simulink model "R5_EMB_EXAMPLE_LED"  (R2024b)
settings: Solver=FixedStepDiscrete  StartTime=0.0  StopTime=S  FixedStep=T  RelTol=1e-3  EnableMultiTasking=on
undefined symbols (not defined in the file): Serial_Port, Standard_Devices, T
libraries: easyio x1

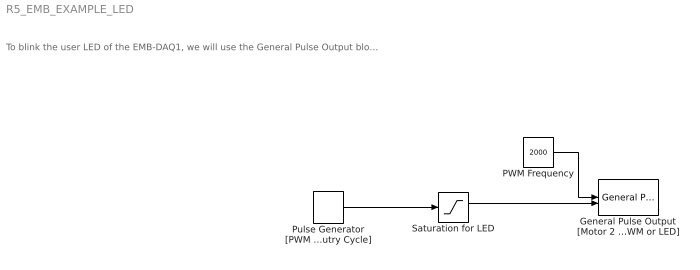
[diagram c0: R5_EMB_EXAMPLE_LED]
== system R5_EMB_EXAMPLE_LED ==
  note: To blink the user LED of the EMB-DAQ1, we will use the General Pulse Output block. The LED is wired to PORT B pin 1. We set the PWM mode to frequency and duty.
  General Pulse Output [Motor 2 - PWM or LED] : easyio/General Pulse Output  SampleTime=T  MaxMissedTicks=10  ShowMissedTicks=0  YieldWhenWaiting=0  DrvName=Standard_Devices/Serial_Port  DrvAddress=6  DrvOptions=[460800 8 0 0 0 0 0 0]  PacketSize=16  DataTypes={'double','double'}  ShowReady=0  ShowError=0  PacketID=1  ByteOrder=1  InitialValue=[0 0]  FinalValue=[0 0]  CfgPrm=N1  PrmCfg=frequency and duty  ResVar=449.8360 Hz - 115156.25 Hz  VarRes=64
  PWM Frequency : Constant  Value=2000  SampleTime=T
  Pulse Generator [PWM % Dutry Cycle] : DiscretePulseGenerator  PulseType=Time based  Period=1  PulseWidth=50
  Saturation for LED : Saturate  UpperLimit=1  LowerLimit=0
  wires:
  Saturation for LED/1 -> General Pulse Output [Motor 2 - PWM or LED]/2
  Pulse Generator [PWM % Dutry Cycle]/1 -> Saturation for LED/1
  PWM Frequency/1 -> General Pulse Output [Motor 2 - PWM or LED]/1
